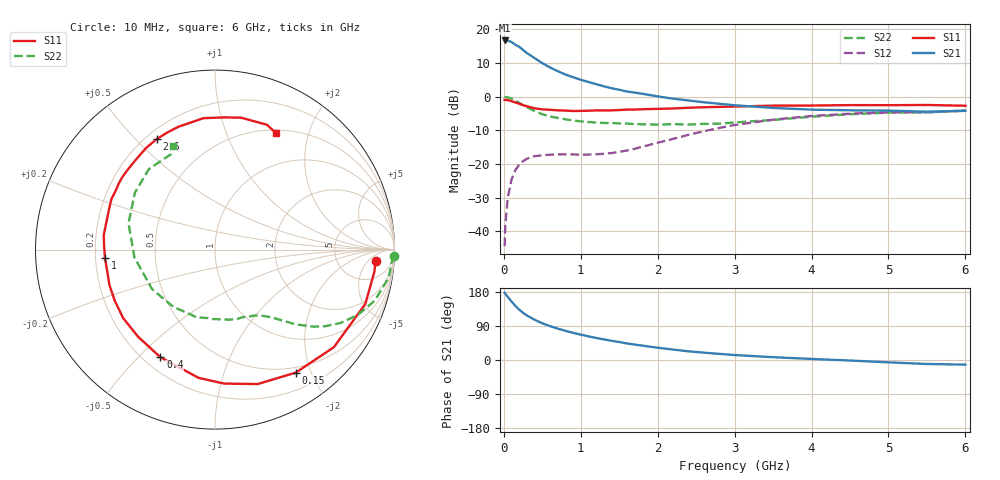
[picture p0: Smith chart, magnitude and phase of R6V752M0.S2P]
! SIEMENS Small Signal Semiconductors
! BFR193
! Si NPN RF Bipolar Junction Transistor in SOT23
! VCE = 0.75 V  IC = 2 mA
! Common Emitter S-Parameters:  May  1996
# GHz  S  MA  R  50
!  f  S11  S21  S12  S22
! GHz  MAG  ANG  MAG  ANG  MAG  ANG  MAG  ANG
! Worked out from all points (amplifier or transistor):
!   36 points, 10 MHz to 6 GHz, reference 50 ohm
!   highest |S21| = 16.7 dB at 10 MHz (marker M1)
!   |S21| within 3 dB of that: start of sweep to 260.6 MHz
!   unconditionally stable (mu >= 1): 1.121 GHz to 2.282 GHz; 5.188 GHz to end of sweep
!   at 250 MHz: K = 0.24, MSG = 16.5 dB, |S12| = -19.2 dB
!   at 1.4 GHz: K = 1.15, MAG = 7.3 dB, |S12| = -16.8 dB
!   at 6 GHz: K = 1.01, MAG = -0.6 dB, |S12| = -4.2 dB
!   S11 on the Smith chart (normalised r, x): 10 MHz: 13, -8; 150 MHz: 0.42, -1.78; 400 MHz: 0.27, -0.58; 1 GHz: 0.24, -0.03; 2.6 GHz: 0.24, +0.58; 6 GHz: 0.54, +1.52
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0.01  0.8976 -4.0  6.848 177.7  0.006 87.6  0.9959 -1.9
0.02  0.8964 -8.0  6.718 174.7  0.0124 85.0  0.9883 -3.7
0.05  0.8905 -19.9  6.782 166.8  0.0308 78.8  0.9799 -9.2
0.1  0.8569 -39.4  6.494 154.4  0.0587 69.2  0.9346 -17.7
0.15  0.8199 -56.7  5.919 142.6  0.0812 60.0  0.8752 -24.6
0.2  0.7859 -72.4  5.502 132.9  0.0978 52.4  0.8087 -30.4
0.25  0.7483 -86.1  4.96 124.4  0.11 46.4  0.7452 -35.0
0.3  0.7204 -97.3  4.453 117.5  0.1196 41.9  0.6962 -38.1
0.4  0.6723 -116.9  3.742 106.3  0.1306 35.0  0.6126 -42.8
0.5  0.6476 -131.4  3.153 96.9  0.1345 30.9  0.5481 -46.3
0.6  0.6384 -143.3  2.717 89.4  0.1375 28.6  0.5082 -48.9
0.8  0.6208 -161.3  2.134 77.1  0.1388 26.8  0.4606 -53.5
1  0.615 -175.8  1.783 66.9  0.1374 29.3  0.4291 -58.8
1.1  0.6182 178.1  1.652 62.4  0.138 31.3  0.4206 -62.1
1.3  0.6236 167.3  1.426 54.4  0.1419 36.5  0.4062 -68.3
1.6  0.6421 153.9  1.193 43.7  0.1585 45.0  0.3983 -79.1
2.2  0.6676 131.2  0.934 27.5  0.2359 53.4  0.3909 -105.0
2.6  0.6964 117.7  0.826 19.4  0.3061 51.3  0.3944 -125.8
3.5  0.7351 95.0  0.68 7.4  0.4557 35.9  0.4509 -174.5
4.5  0.7493 78.7  0.627 -1.4  0.559 16.6  0.5476 144.5
5.5  0.7531 67.4  0.598 -10.5  0.5861 -0.2  0.5855 114.7
6  0.733 62.3  0.619 -12.3  0.6164 -5.0  0.6226 112.1
